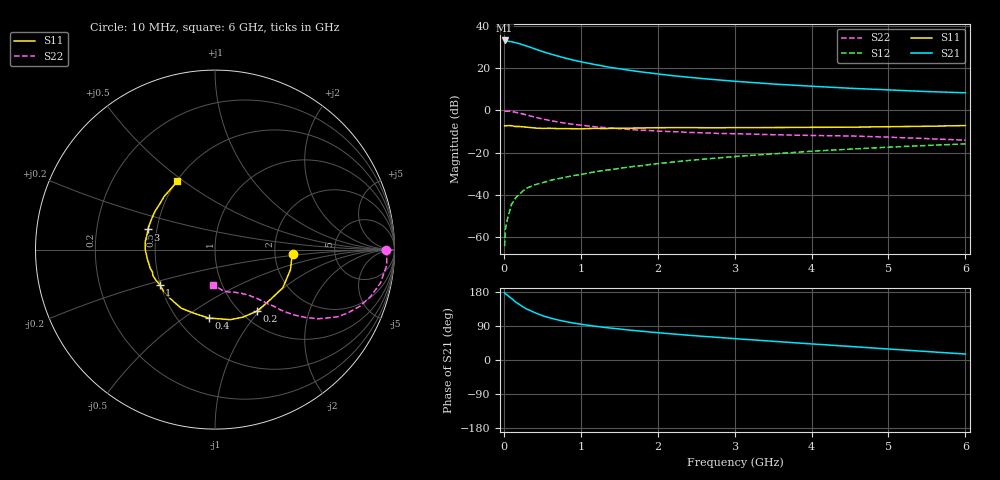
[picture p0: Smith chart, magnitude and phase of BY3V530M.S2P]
! SIEMENS Small Signal Semiconductors
! BFY420
! Si NPN RF SIEGET Grounded Emitter Transistor in MICRO-X
! VCE = 3.5 V  IC = 30 mA
! Common Emitter S-Parameters:  October  1996
# GHz  S  MA  R  50
!  f  S11  S21  S12  S22
! GHz  MAG  ANG  MAG  ANG  MAG  ANG  MAG  ANG
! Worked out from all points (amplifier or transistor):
!   36 points, 10 MHz to 6 GHz, reference 50 ohm
!   highest |S21| = 33.2 dB at 10 MHz (marker M1)
!   |S21| within 3 dB of that: start of sweep to 323.8 MHz
!   unconditionally stable (mu >= 1): start of sweep to 11.97 MHz; 1.713 GHz to end of sweep
!   at 250 MHz: K = 0.36, MSG = 34.6 dB, |S12| = -38.2 dB
!   at 1.4 GHz: K = 0.96, MSG = 24.2 dB, |S12| = -28.1 dB
!   at 6 GHz: K = 1.06, MAG = 10.7 dB, |S12| = -15.9 dB
!   S11 on the Smith chart (normalised r, x): 10 MHz: 2.52, -0.14; 200 MHz: 1.17, -0.97; 400 MHz: 0.70, -0.63; 1 GHz: 0.50, -0.22; 3 GHz: 0.45, +0.12; 6 GHz: 0.50, +0.48
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0.01  0.4328 -3.0  45.67 178.0  0.0006 113.2  0.9503 -0.1
0.02  0.4307 -5.9  45.42 175.0  0.0015 88.8  0.9575 -1.4
0.1  0.4334 -29.4  42.59 162.3  0.0059 79.6  0.9402 -11.4
0.15  0.415 -42.9  40.5 153.5  0.0082 73.6  0.905 -16.9
0.2  0.4151 -55.9  38.38 146.9  0.0102 72.7  0.8665 -21.4
0.25  0.4072 -67.6  35.84 139.9  0.0123 68.2  0.8196 -25.5
0.3  0.3997 -77.6  33.47 134.3  0.0143 68.2  0.7782 -28.8
0.4  0.3828 -95.3  28.95 125.2  0.0172 64.9  0.6944 -33.7
0.5  0.3736 -109.2  24.97 117.1  0.0191 62.8  0.6276 -37.0
0.6  0.3766 -120.1  22.01 111.1  0.0218 62.8  0.5745 -39.4
0.7  0.3702 -128.9  19.53 105.9  0.0238 62.2  0.5319 -41.2
0.8  0.3697 -136.1  17.4 101.5  0.026 61.0  0.4963 -42.6
1  0.3651 -147.7  14.29 94.4  0.03 63.3  0.4458 -44.4
1.1  0.3708 -152.8  13.16 91.5  0.0328 62.6  0.425 -45.6
1.4  0.3758 -163.9  10.37 84.0  0.0393 63.4  0.3817 -47.8
1.6  0.3784 -169.8  9.122 79.6  0.0446 63.1  0.3559 -49.5
2.2  0.3901 176.6  6.658 68.7  0.0596 60.9  0.3132 -54.3
3  0.3908 163.3  4.917 56.4  0.0804 56.4  0.2804 -60.3
3.5  0.3919 155.3  4.231 49.4  0.0931 53.2  0.265 -64.2
4.5  0.3994 140.3  3.352 35.8  0.1205 44.9  0.247 -72.8
5.5  0.4201 125.0  2.8 22.4  0.1474 35.9  0.214 -85.2
6  0.4366 118.6  2.618 15.7  0.1606 31.0  0.1966 -93.2
